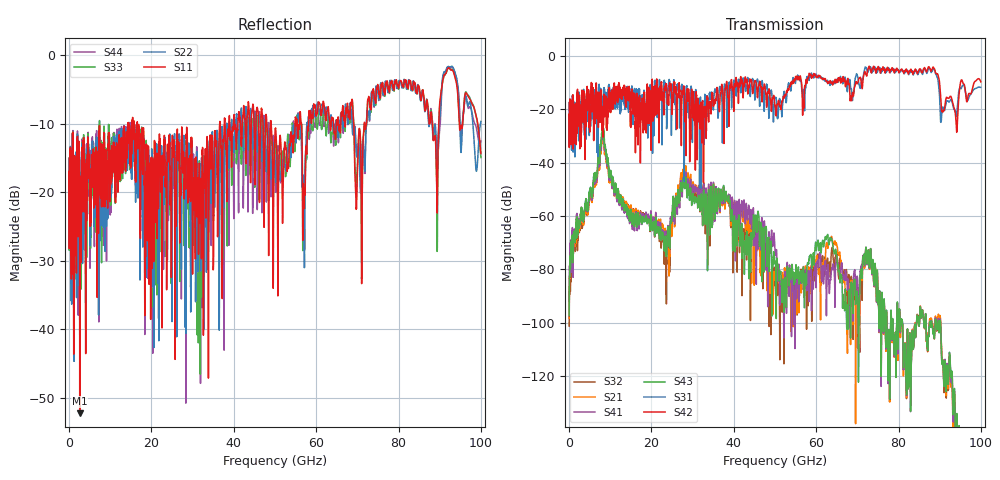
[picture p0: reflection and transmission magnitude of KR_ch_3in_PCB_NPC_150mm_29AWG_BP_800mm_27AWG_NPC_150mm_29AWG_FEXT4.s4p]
# GHz S RI R 45
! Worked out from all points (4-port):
!   4000 points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, 25 MHz to 100 GHz, reference 45 ohm
!   strongest paths, dB at 25 MHz, 25.02 GHz, 50.02 GHz, 75.03 GHz, 100 GHz:
!     S42: -22.2, -20.8, -18.7, -4.1, -9.8
!     S31: -22.1, -12.7, -15.7, -5.1, -11.8
!     S43: -97.3, -59.3, -77.7, -90.8, -170.5
!     S41: -91.9, -59.3, -73.1, -91.0, -168.4
!     S21: -98.2, -63.8, -82.5, -91.1, -168.6
!     S32: -101.2, -60.8, -86.1, -90.7, -167.1
!   lowest |S11| = -52.2 dB at 2.6 GHz (marker M1), VSWR 1.00, Z = 45.1 + j0.18 ohm
!   |S11| at or under -10 dB: start of sweep to 14.33 GHz; 16.58 GHz to 36.61 GHz (20.03 GHz wide, 75.3 % of centre); 49.07 GHz to 54.89 GHz (5.823 GHz wide, 11.2 % of centre)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
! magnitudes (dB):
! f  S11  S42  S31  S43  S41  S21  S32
! 25 MHz  -17.4  -22.2  -22.1  -97.3  -91.9  -98.2  -101.2
! 2.6 GHz  -52.2  -27.8  -31.5  -63.3  -63.3  -64.8  -65.3
! 8.1 GHz  -13.0  -19.0  -19.2  -27.5  -29.5  -31.1  -29.0
! 23.4 GHz  -18.1  -12.9  -12.9  -68.2  -66.3  -65.6  -71.6
! 28.02 GHz  -18.5  -13.2  -24.0  -49.3  -47.9  -45.8  -47.4
! 49.15 GHz  -10.7  -20.6  -13.0  -71.5  -65.6  -81.1  -81.9
! 100 GHz  -14.4  -9.8  -11.8  -170.5  -168.4  -168.6  -167.1
